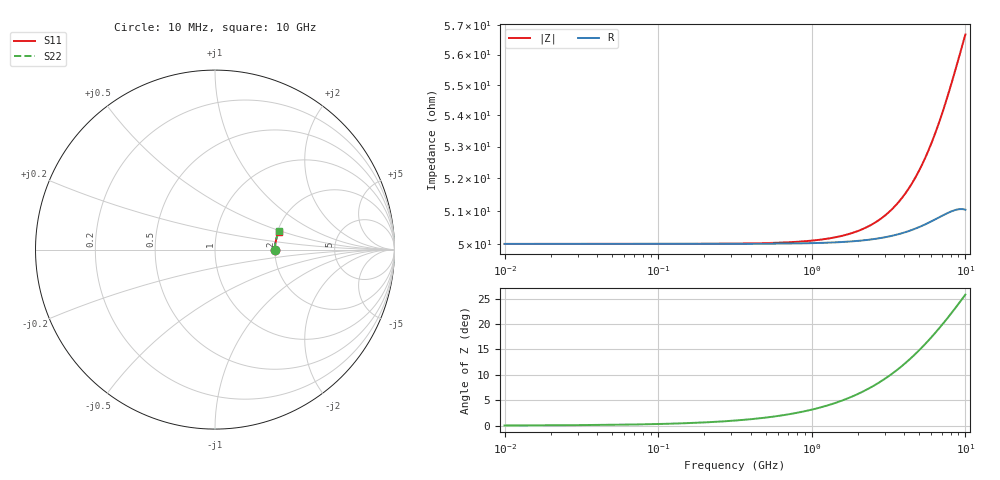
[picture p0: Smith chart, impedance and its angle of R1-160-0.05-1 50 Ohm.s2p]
!version-2
!date-03.2021
# MHz S RI R 50
!Freq ReS11 ImS11 ReS21 ImS21 ReS12 ImS12 ReS22 ImS22
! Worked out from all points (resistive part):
!   501 points, 10 MHz to 10 GHz, reference 50 ohm
!   read as one part in series: R = 50 ohm at 50 MHz
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10  0.3333 0.000118  0.6667 -0.000125  0.6667 -0.000125  0.3333 0.00012
50  0.3333 0.000588  0.6667 -0.000625  0.6667 -0.000625  0.3333 0.000599
450  0.3334 0.00529  0.6666 -0.00562  0.6666 -0.00562  0.3334 0.00539
850  0.3336 0.00998  0.6664 -0.0106  0.6664 -0.0106  0.3336 0.0102
1270  0.3339 0.0149  0.6661 -0.0158  0.6661 -0.0158  0.3339 0.0152
1690  0.3342 0.0198  0.6657 -0.021  0.6657 -0.021  0.3343 0.0201
2090  0.3347 0.0244  0.6652 -0.0259  0.6652 -0.0259  0.3348 0.0248
2510  0.3353 0.0292  0.6646 -0.031  0.6646 -0.031  0.3354 0.0297
2930  0.336 0.0339  0.6639 -0.0361  0.6639 -0.0361  0.3361 0.0346
3350  0.3368 0.0386  0.6631 -0.0411  0.6631 -0.0411  0.337 0.0393
3750  0.3376 0.043  0.6623 -0.0458  0.6623 -0.0458  0.3378 0.0438
4150  0.3385 0.0473  0.6613 -0.0504  0.6613 -0.0504  0.3388 0.0482
4570  0.3396 0.0518  0.6603 -0.0551  0.6603 -0.0551  0.3398 0.0528
5010  0.3407 0.0564  0.6591 -0.06  0.6591 -0.06  0.341 0.0574
5850  0.343 0.0648  0.6568 -0.0691  0.6568 -0.0691  0.3435 0.0661
6670  0.3454 0.0727  0.6543 -0.0776  0.6543 -0.0776  0.346 0.0741
7090  0.3466 0.0766  0.653 -0.0818  0.653 -0.0818  0.3473 0.0781
7510  0.3479 0.0803  0.6517 -0.0858  0.6517 -0.0858  0.3486 0.0819
8350  0.3503 0.0876  0.6492 -0.0937  0.6492 -0.0937  0.3513 0.0893
9230  0.3527 0.0948  0.6467 -0.1015  0.6467 -0.1015  0.3539 0.0966
9810  0.3542 0.0993  0.6451 -0.1064  0.6451 -0.1064  0.3555 0.1013
10000  0.3546 0.1007  0.6447 -0.108  0.6447 -0.108  0.356 0.1027
